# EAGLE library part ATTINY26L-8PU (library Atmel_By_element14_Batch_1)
Microcontroller
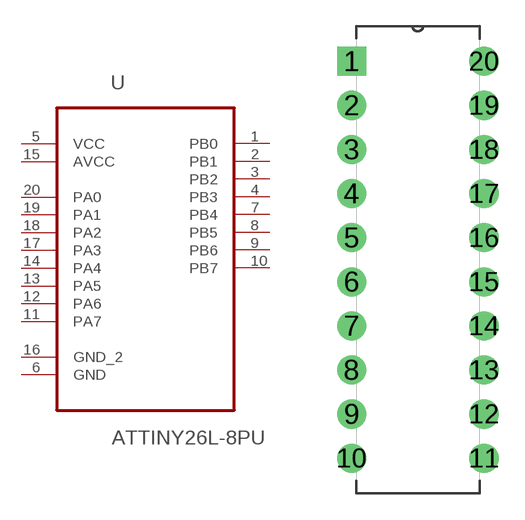
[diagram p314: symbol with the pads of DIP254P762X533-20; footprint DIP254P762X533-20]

Designator prefix U

## ATTINY26L-8PU (MPN: ATTINY26L-8PU; OC_FARNELL: 9171657; OC_NEWARK: 01M6920; PACKAGE: DIP-20; SUPPLIER: ATMEL)  [DIP254P762X533-20]
1  PB0
2  PB1
3  PB2
4  PB3
5  VCC  pwr
6  GND  pas
7  PB4
8  PB5
9  PB6
10  PB7
11  PA7
12  PA6
13  PA5
14  PA4
15  AVCC  pwr
16  GND_2  pas
17  PA3
18  PA2
19  PA1
20  PA0

## Footprint DIP254P762X533-20 (pad centres in mm)
drill 1.118 square: 1 -7.62,22.86
drill 1.118: 2 -7.62,20.32; 3 -7.62,17.78; 4 -7.62,15.24; 5 -7.62,12.7; 6 -7.62,10.16; 7 -7.62,7.62; 8 -7.62,5.08; 9 -7.62,2.54; 10 -7.62,0; 11 0,0; 12 0,2.54; 13 0,5.08; 14 0,7.62; 15 0,10.16; 16 0,12.7; 17 0,15.24; 18 0,17.78; 19 0,20.32; 20 0,22.86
